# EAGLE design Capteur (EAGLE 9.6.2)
COMPANY: Adafruit Industries; DRAWN: KTOWN; REV: A
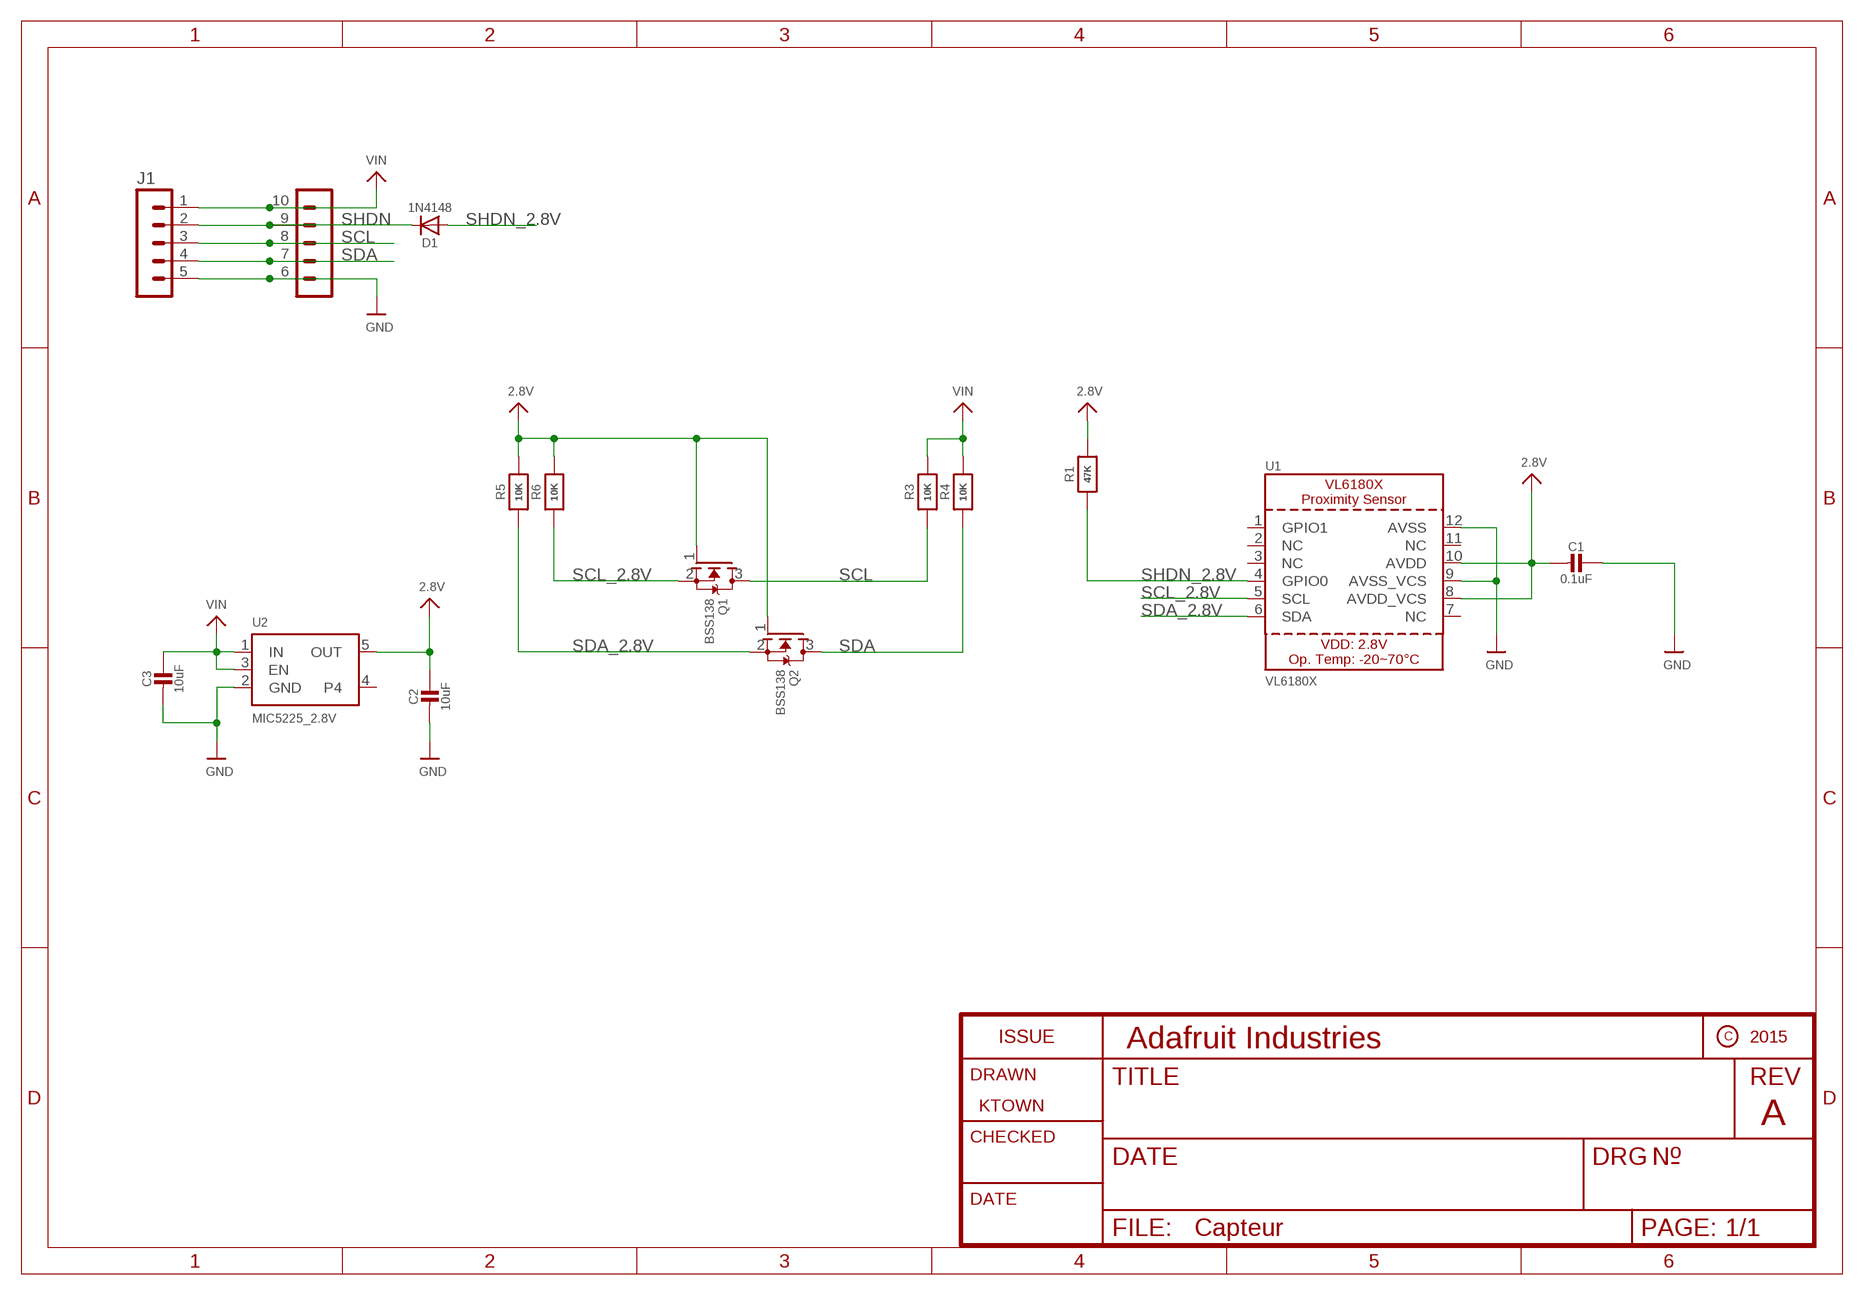
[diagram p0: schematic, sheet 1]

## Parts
C1  0.1uF  CAP_CERAMIC0805-NOOUTLINE  [0805-NO]
C2  10uF  CAP_CERAMIC0805-NOOUTLINE  [0805-NO]
C3  10uF  CAP_CERAMIC0805-NOOUTLINE  [0805-NO]
D1  1N4148  DIODESOD-323  [SOD-323]
J1  CON5X2  [PA10]
Q1  BSS138  MOSFET-NWIDE  [SOT23-WIDE]
Q2  BSS138  MOSFET-NWIDE  [SOT23-WIDE]
R1  47K  RESISTOR0805_NOOUTLINE  [0805-NO]
R3  10K  RESISTOR0805_NOOUTLINE  [0805-NO]
R4  10K  RESISTOR0805_NOOUTLINE  [0805-NO]
R5  10K  RESISTOR0805_NOOUTLINE  [0805-NO]
R6  10K  RESISTOR0805_NOOUTLINE  [0805-NO]
U1  VL6180X  [VL6180]
U2  MIC5225_2.8V  VREG_SOT23-5  [SOT23-5]

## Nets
2.8V: C1.2 C2.1 Q1.1(G) Q2.1(G) R1.2 R5.2 R6.2 U1.8(AVDD_VCS) U1.10(AVDD) U2.5(OUT)
GND: C1.1 C2.2 C3.2 J1.5 J1.6 U1.9(AVSS_VCS) U1.12(AVSS) U2.2(GND)
SCL: J1.3 J1.8 Q1.3(D) R3.1
SCL_2.8V: Q1.2(S) R6.1 U1.5(SCL)
SDA: J1.4 J1.7 Q2.3(D) R4.1
SDA_2.8V: Q2.2(S) R5.1 U1.6(SDA)
SHDN: D1.C J1.2 J1.9
SHDN_2.8V: D1.A R1.1 U1.4(GPIO0)
VIN: C3.1 J1.1 J1.10 R3.2 R4.2 U2.1(IN) U2.3(EN)
Unconnected: U1.1(GPIO1) U1.2(NC) U1.3(NC) U1.7(NC) U1.11(NC) U2.4

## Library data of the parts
C1-C3 = microbuilder:CAP_CERAMIC: Ceramic Capacitors
D1 = microbuilder:DIODE: Diode
J1 = 0IUT xPROJETS (1):CON5X2
Q1 Q2 = microbuilder:MOSFET-N: N-Channel Mosfet LEGEND VDS: Voltage Drain-Source ID: Drain Current RDS(ON): Drain-Source On-State Resistance VGS(TH): Gate-Source Threshold Voltage CISS: Drain-Source Input Capacitance SOT-23 Name VDS ID RDS(ON) VGS(TH) CISS Order Number 2N7002E 60V 260mA 2.5 Ohm 2.5V @ 250uA 26.7pF @ 25V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
R1 R3-R6 = microbuilder:RESISTOR: Resistors
U1 = microbuilder:VL6180X: VL6180x Proximity and Light Sensor with Gesture Recognition Supply Level: 2.8V (3.0V Max!) Range: 0-10cm Light Sensor: 0..100K Lux (16-bit output) IR emitter: 850 nm I2C Address: 0x29 (7-bit)
U2 = microbuilder:VREG_SOT23-5: SOT23-5 Fixed Voltage Regulators Part Current Out V Out V In V Dropout θJA (°C/W) TJ (°C) Digikey Part No. ADP121 150mA 3.3V 3.4-5.5V 0.09V @ 150mA -- -- ADP121-AUJZ33R7CT-ND ADP121 150mA 3.0V 3.1-5.5V 0.09V @ 150mA -- -- ADP121-AUJZ30R7CT-ND ADP122 300mA 3.3V 3.4-5.5V 0.085V @ 300mA -- --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

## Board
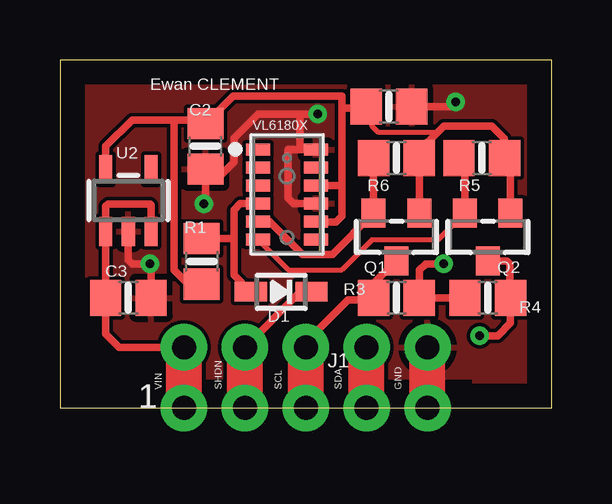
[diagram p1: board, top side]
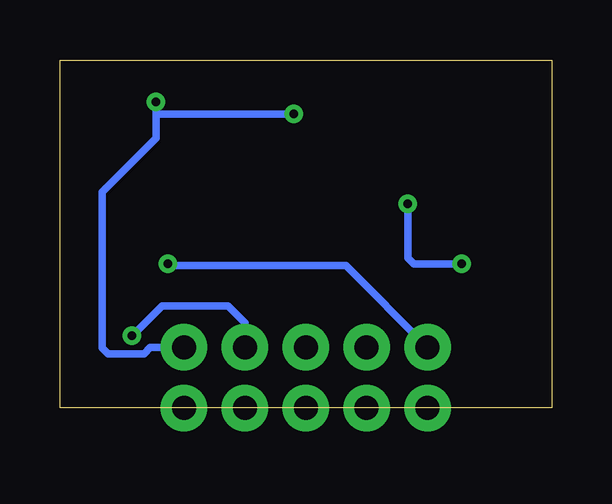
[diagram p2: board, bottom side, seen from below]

Size 20.5 x 14.5 mm. Coordinates in mm from the lower left corner, seen from the top.
Outline: 0,0 20.5,0 20.5,14.5 0,14.5 0,0
Copper layers (1*16): Top 0.035mm / dielectric 1.5mm / Bottom 0.035mm
Design rules "default": minimum track width 6mil, minimum drill 0.35mm, track to track 6mil, track to pad 6mil, pad to pad 6mil, via to via 6mil, smd to smd 6mil, copper to edge 40mil, drill to drill 6mil, minimum pad ring 10mil, minimum via ring 8mil, stop-mask expansion 4mil, vias tented up to drill 0mil, thermal gap 10mil

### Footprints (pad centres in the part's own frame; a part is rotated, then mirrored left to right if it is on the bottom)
0805-NO = smd 1.3 x 1.5: 1 -0.95,0; 2 0.95,0
SOD-323 = smd 1.35 x 0.8: A 1.27,0; C -1.27,0
PA10 = drill 1 pad 1.93: 1 -5.08,-1.27; 2 -2.54,-1.27; 3 0,-1.27; 4 2.54,-1.27; 5 5.08,-1.27; 6 5.08,1.27; 7 2.54,1.27; 8 0,1.27; 9 -2.54,1.27; 10 -5.08,1.27
SOT23-WIDE = smd 1 x 1.2: 1 -0.95,-1; 2 0.95,-1; 3 0,1
VL6180 = smd 1 x 0.5: 1 -1.2,1.875; 2 -1.2,1.125; 3 -1.2,0.375; 4 -1.2,-0.375; 5 -1.2,-1.125; 6 -1.2,-1.875; 7 1.2,-1.875; 8 1.2,-1.125; 9 1.2,-0.375; 10 1.2,0.375; 11 1.2,1.125; 12 1.2,1.875
SOT23-5 = smd 0.55 x 1.2: 1 -0.95,-1.3; 2 0,-1.3; 3 0.95,-1.3; 4 0.95,1.3; 5 -0.95,1.3

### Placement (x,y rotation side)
C1  13.72,12.55 180 top
C2  6.07,10.9 270 top
C3  2.85,4.58 0 top
D1  9.22,4.83 180 top
J1  10.25,1.25 0 top
Q1  14.03,7.12 180 top
Q2  17.84,7.12 180 top
R1  5.91,6.1 270 top
R3  14.03,4.58 0 top
R4  17.84,4.58 180 top
R5  17.59,10.41 0 top
R6  14.03,10.41 0 top
U1  9.47,8.89 0 top
U2  2.85,8.64 0 top

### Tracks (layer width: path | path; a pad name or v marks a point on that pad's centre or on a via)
2.8V
  Top 0.152: R6.2 14.98,10.73 | 10.69,7.75 U1.8
  Top 0.203: 15.75,11.5 13.25,11.5 13,11.75 13,12.32 C1.2
  Top 0.305: 14.98,10.73 15.75,11.5 16,11.75 18,11.75 18.54,11.21 R5.2 18.79,10.16 Q2.1 | Q1.1 R6.2 | 11.75,9.27 U1.10 | 10.69,7.75 11.5,7.75 11.75,8 11.75,9.27 | U2.5 1.9,10.9 3,12 4.75,12 | 4.75,12 5.92,12 C2.1 7.21,13 11.75,13 11.75,12.5 | 4.75,12 4.75,5.75 5.35,5.15 R1.2 | 11.75,9.27 11.75,12.5 | C1.2 12.72,12.5 11.75,12.5
GND  (via drill 0.35)
  Top 0.152: 6.07,8.56 v6,8.5 | v3.75,6 3.8,5.95
  Top 0.305: C2.2 6.07,9.75 | 6.07,9.75 6.07,8.56 | 3.8,5.95 C3.2 | v10.75,12.25 10,12.25 | 10,12.25 8.25,12.25 7.25,11.25 7.25,10.25 6.75,9.75 6.07,9.75 | U1.12 10,10.77 | 10,10.77 10,12.25 | U1.9 9.73,8.52 9.5,8.75 9.5,10.75 9.52,10.77 10,10.77 | v3.75,6 3,6 2.85,6.15 U2.2 | v16.5,12.75 16.3,12.55 C1.1
  Top 1.5: J1.5 J1.6
  Bottom 0.305: v6,8.5 6,6.25 5.75,6 v3.75,6 | J1.6 16.73,2.52 17,2.25 18.5,2.25 18.75,2.5 18.75,9 16.5,11.25 16.5,12.25 | 16.5,12.25 v16.5,12.75 | v10.75,12.25 16.5,12.25
  pour Top: 0,0 0,14.5 20.5,14.5 20.5,0 17.25,0 17.25,1.25 3,1.25 3,0
SCL
  Top 0.152: 13.08,4.5 R3.1 13.08,5.17 | 10.25,2.75 J1.8
  Top 0.305: 13.08,5.17 Q1.3 | 13.08,4.5 12,4.5 10.25,2.75
  Top 1.5: J1.3 J1.8
SCL_2.8V
  Top 0.305: R6.1 Q1.2 11.36,6.39 10.11,6.39 8.73,7.76 U1.5
SDA  (via drill 0.35)
  Top 0.152: R4.1 18.75,4.62
  Top 0.305: R4.1 18.79,3.54 18.25,3 v17.5,3 | 18.75,4.62 18.75,6 18.63,6.12 Q2.3
  Top 1.5: J1.4 J1.7
  Bottom 0.305: v17.5,3 16.25,4.25 13.5,4.25 12.79,3.54 J1.7
SDA_2.8V
  Top 0.152: 16.89,10.16 R5.1 | 9.52,5.76 9.52,5.75
  Top 0.203: Q2.2 15.77,7 13,7 11.75,5.75 9.52,5.75 | U1.6 9.52,5.76
  Top 0.305: Q2.2 16.89,10.16
SHDN
  Top 0.305: D1.C 10.02,4.83 J1.9
  Top 1.5: J1.2 J1.9
SHDN_2.8V
  Top 0.305: D1.A 7.25,5.53 7.25,7 | 7.25,7 7.25,8.25 7.51,8.52 U1.4 | 7.25,7 7.2,7.05 R1.1
VIN  (via drill 0.35)
  Top 0.305: U2.3 3.8,8.45 3.75,8.5 2,8.5 1.9,8.4 U2.1 C3.1 1.9,3.08 2.46,2.52 J1.10 | R4.2 R3.2 14.98,5.73 15.25,6 v16,6
  Top 1.5: J1.1 J1.10
  Bottom 0.305: v16,6 15.92,5.92 8.57,5.92 J1.10

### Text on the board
tNames: Ewan CLEMENT | VIN | SHDN | SCL | SDA | GND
